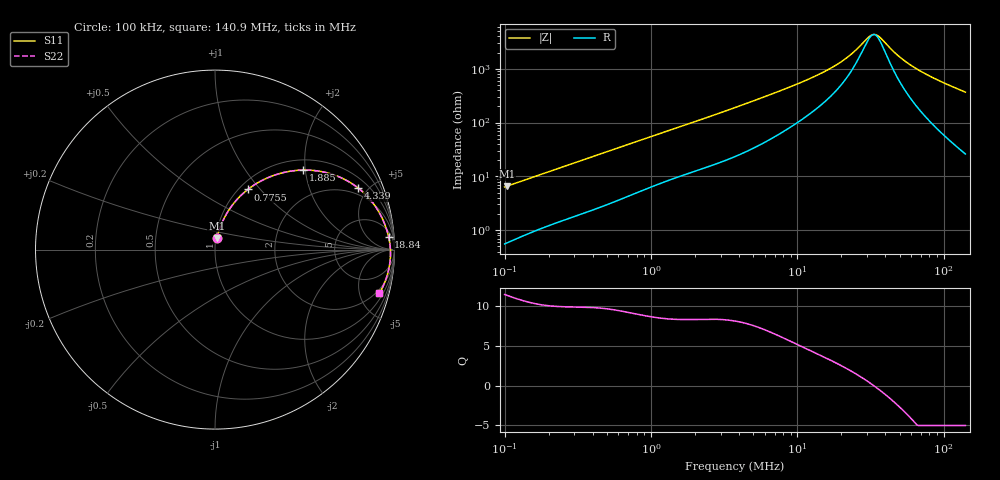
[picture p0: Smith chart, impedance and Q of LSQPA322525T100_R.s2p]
! LSQPA322525T100_R  S-PARAMETER MODEL  ( General Type )
! Model Generated by TAIYO YUDEN Corporation (http://www.ty-top.com)
! Version 2.0
! TAIYO YUDEN Control No. 100810NF25SB-FKC
! Copyright(c) 2007 TAIYO YUDEN CO.,LTD. All Rights Reserved.
! Product Description (link to TY-COMPAS)
! https://ds.yuden.co.jp/TYCOMPAS/or/detail?pn=LSQPA322525T100KR&u=M
! Products Name : Inductors
! Characteristics :
!  Inductance : 10 uH , SRF(min) : 23 MHz , DC Resistance(max) : 0.1729 Ohm
!  Rated Current : Saturation :900 mA , Temp Rise : 900 mA (40 degC)
!  Case Size : 3.2 x 2.5 / 0.126 x 0.098 [mm/inch] , Thickness : 2.5 / 0.098 [mm/inch]
!  (Conditions: Temperature = 25 degC , DC Bias Current/Voltage = 0A / 0V)
! External Node Assignments :
!  1  o---GGG---o  2
! GND o---------o GND
! Frequency Range : 0.1MHz  -  140.89697MHz  [ 402 STEP ]
# MHz S RI R 50
! Freq[MHz].  S11 Real  S11 Imag  S21 Real  S21 Imag  S12 Real  S12 Imag  S22 Real  S22 Imag
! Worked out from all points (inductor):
!   401 points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, 100 kHz to 140.9 MHz, reference 50 ohm
!   read as one part in series: L = 9.92 uH near 103.7 kHz
!   highest Q = 11.3 at 103.7 kHz (marker M1), where L = 10 uH
!   self-resonance near 33.23 MHz
!   S11 on the Smith chart (normalised r, x): 100 kHz: 1.01, +0.13; 775.5 kHz: 1.10, +0.86; 1.885 MHz: 1.24, +1.95; 4.339 MHz: 1.55, +4.34; 18.84 MHz: 9, +23; 140.9 MHz: 1.52, -7.34
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0.1  0.00944 0.0623  0.9906 -0.0623  0.9906 -0.0623  0.00944 0.0623
0.103692  0.00996 0.0644  0.99 -0.0644  0.99 -0.0644  0.00996 0.0644
0.336853  0.0548 0.1824  0.9452 -0.1824  0.9452 -0.1824  0.0548 0.1824
0.775469  0.1834 0.3354  0.8166 -0.3354  0.8166 -0.3354  0.1834 0.3354
1.134703  0.2964 0.4014  0.7036 -0.4014  0.7036 -0.4014  0.2964 0.4014
1.884973  0.4929 0.4431  0.5071 -0.4431  0.5071 -0.4431  0.4929 0.4431
2.612196  0.6269 0.4272  0.3731 -0.4272  0.3731 -0.4272  0.6269 0.4272
3.753625  0.7567 0.3716  0.2433 -0.3716  0.2433 -0.3716  0.7567 0.3716
4.339392  0.7988 0.3422  0.2012 -0.3422  0.2012 -0.3422  0.7988 0.3422
6.951963  0.8941 0.2401  0.1059 -0.2401  0.1059 -0.2401  0.8941 0.2401
12.64421  0.95 0.1303  0.05 -0.1303  0.05 -0.1303  0.95 0.1303
18.84002  0.9671 0.0726  0.0329 -0.0726  0.0329 -0.0726  0.9671 0.0726
23.41793  0.9727 0.0442  0.0273 -0.0442  0.0273 -0.0442  0.9727 0.0442
30.18284  0.9766 0.0122  0.0234 -0.0122  0.0234 -0.0122  0.9766 0.0122
32.45257  0.9773 0.00301  0.0227 -0.00301  0.0227 -0.00301  0.9773 0.00301
34.26619  0.9776 -0.00388  0.0224 0.00388  0.0224 0.00388  0.9776 -0.00388
36.18117  0.9778 -0.0108  0.0222 0.0108  0.0222 0.0108  0.9778 -0.0108
42.59248  0.9778 -0.0321  0.0222 0.0321  0.0222 0.0321  0.9778 -0.0321
52.94195  0.9757 -0.062  0.0243 0.062  0.0243 0.062  0.9757 -0.062
68.23567  0.9699 -0.1004  0.0301 0.1004  0.0301 0.1004  0.9699 -0.1004
96.29069  0.9535 -0.1614  0.0465 0.1614  0.0465 0.1614  0.9535 -0.1614
140.897  0.9162 -0.2438  0.0838 0.2438  0.0838 0.2438  0.9162 -0.2438
